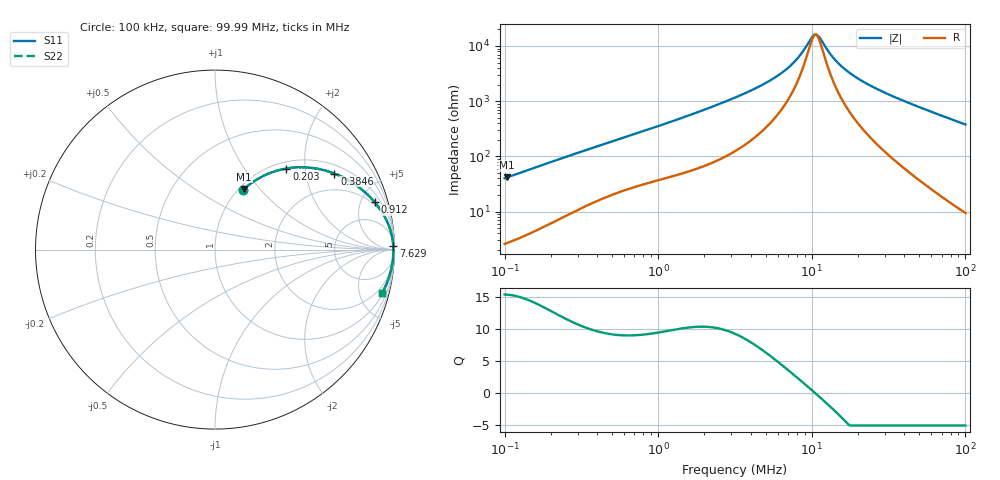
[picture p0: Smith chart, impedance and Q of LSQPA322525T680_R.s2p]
! LSQPA322525T680_R  S-PARAMETER MODEL  ( General Type )
! Model Generated by TAIYO YUDEN Corporation (http://www.ty-top.com)
! Version 2.0
! TAIYO YUDEN Control No. 100810NF25SB-FAC
! Copyright(c) 2007 TAIYO YUDEN CO.,LTD. All Rights Reserved.
! Product Description (link to TY-COMPAS)
! https://ds.yuden.co.jp/TYCOMPAS/or/detail?pn=LSQPA322525T680KR&u=M
! Products Name : Inductors
! Characteristics :
!  Inductance : 68 uH , SRF(min) : 8.0 MHz , DC Resistance(max) : 1.3 Ohm
!  Rated Current : Saturation :320 mA , Temp Rise : 410 mA (40 degC)
!  Case Size : 3.2 x 2.5 / 0.126 x 0.098 [mm/inch] , Thickness : 2.5 / 0.098 [mm/inch]
!  (Conditions: Temperature = 25 degC , DC Bias Current/Voltage = 0A / 0V)
! External Node Assignments :
!  1  o---GGG---o  2
! GND o---------o GND
! Frequency Range : 0.1MHz  -  99.992428MHz  [ 402 STEP ]
# MHz S RI R 50
! Freq[MHz].  S11 Real  S11 Imag  S21 Real  S21 Imag  S12 Real  S12 Imag  S22 Real  S22 Imag
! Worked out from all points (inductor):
!   401 points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, 100 kHz to 99.99 MHz, reference 50 ohm
!   read as one part in series: L = 63.3 uH near 103.5 kHz
!   highest Q = 15.4 at 103.5 kHz (marker M1), where L = 63.5 uH
!   self-resonance near 10.41 MHz
!   S11 on the Smith chart (normalised r, x): 100 kHz: 1.05, +0.80; 203 kHz: 1.12, +1.59; 384.6 kHz: 1.30, +2.91; 912 kHz: 1.69, +6.43; 7.629 MHz: open; 99.99 MHz: 1.19, -7.55
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0.1  0.1535 0.3295  0.8465 -0.3295  0.8465 -0.3295  0.1535 0.3295
0.103514  0.1618 0.3373  0.8382 -0.3373  0.8382 -0.3373  0.1618 0.3373
0.203  0.3975 0.4518  0.6025 -0.4518  0.6025 -0.4518  0.3975 0.4518
0.318049  0.5912 0.4464  0.4088 -0.4464  0.4088 -0.4464  0.5912 0.4464
0.384586  0.6651 0.4238  0.3349 -0.4238  0.3349 -0.4238  0.6651 0.4238
0.582092  0.7953 0.3522  0.2047 -0.3522  0.2047 -0.3522  0.7953 0.3522
0.911989  0.8894 0.2647  0.1106 -0.2647  0.1106 -0.2647  0.8894 0.2647
1.011554  0.9051 0.2452  0.0949 -0.2452  0.0949 -0.2452  0.9051 0.2452
1.85134  0.9633 0.1461  0.0367 -0.1461  0.0367 -0.1461  0.9633 0.1461
3.162158  0.9838 0.0836  0.0162 -0.0836  0.0162 -0.0836  0.9838 0.0836
5.401085  0.9914 0.0403  0.00864 -0.0403  0.00864 -0.0403  0.9914 0.0403
6.531006  0.9926 0.028  0.00743 -0.028  0.00743 -0.028  0.9926 0.028
7.629206  0.9932 0.0186  0.00678 -0.0186  0.00678 -0.0186  0.9932 0.0186
8.609517  0.9936 0.0116  0.00644 -0.0116  0.00644 -0.0116  0.9936 0.0116
10.05722  0.9938 0.00287  0.00619 -0.00287  0.00619 -0.00287  0.9938 0.00287
10.592  0.9939 -3.32e-05  0.00615 3.32e-05  0.00615 3.32e-05  0.9939 -3.32e-05
10.96422  0.9939 -0.00197  0.00613 0.00197  0.00613 0.00197  0.9939 -0.00197
13.96293  0.9937 -0.0157  0.00627 0.0157  0.00627 0.0157  0.9937 -0.0157
17.47734  0.9932 -0.0292  0.00683 0.0292  0.00683 0.0292  0.9932 -0.0292
22.6451  0.9919 -0.0467  0.00813 0.0467  0.00813 0.0467  0.9919 -0.0467
31.98693  0.9884 -0.0749  0.0116 0.0749  0.0116 0.0749  0.9884 -0.0749
99.99243  0.9292 -0.2443  0.0708 0.2443  0.0708 0.2443  0.9292 -0.2443
